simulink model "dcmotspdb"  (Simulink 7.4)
settings: Solver=ode15s  StartTime=0.0  StopTime=0.1  MaxStep=2e-5  RelTol=1e-5

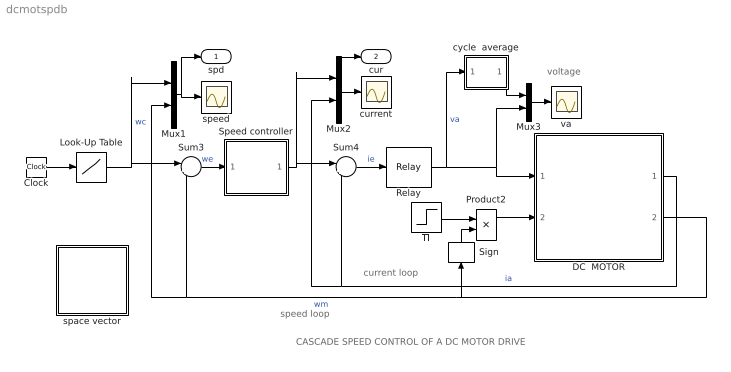
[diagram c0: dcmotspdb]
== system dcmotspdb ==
  note: voltage
  note: speed loop
  note: current loop
  note: CASCADE SPEED CONTROL OF A DC MOTOR DRIVE
  Clock : Clock
  DC  MOTOR : Subsystem  mask{Ra=2, La=0.0052, J=1.5e-4, Bm=1e-3, K=0.1}
      mask prompts: Ra "Armature resistance [ohm]"; La "Armature inductance [H]"; J "Moment of inertia [Kg.m^2]"; Bm "Frictional torque cefficient"; K "Electromechanical coupling coefficient [N.m/A]"
      mask help: Dynamic model of a dc motor
  Look-Up Table : Lookup  InputValues=[0 .03 .03 .08]  Table=[100 100 -100 -100]  OutDataType=sfix(16)  OutScaling=2^0
  Mux1 : Mux  Inputs=2
  Mux2 : Mux  Inputs=2
  Mux3 : Mux  Inputs=2
  Product2 : Product  OutDataType=sfix(16)  OutScaling=2^0
  Relay : Relay  OnSwitchValue=2  OffSwitchValue=-2  OnOutputValue=60  OffOutputValue=-60  OutDataType=sfix(16)  OutScaling=2^0
  Sign : Signum
  Speed controller : Subsystem  mask{Kp=1.5, Ki=650, sat=18}
      mask prompts: Kp "Proportional gain (Kp)"; Ki "Integral gain (Ki)"; sat "Saturation limit [pu]"
      mask help: Proportional-Integral Speed Controller
  Sum3 : Sum  Inputs=|+-  OutDataType=sfix(16)  OutScaling=2^0
  Sum4 : Sum  Inputs=|+-  OutDataType=sfix(16)  OutScaling=2^0
  Tl : Step  Time=0.07  SampleTime=0
  current : Scope
  cycle  average : Subsystem
  space vector : Subsystem
  speed : Scope
  va : Scope
  spd : Outport
  cur : Outport  Port=2
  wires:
  Mux1/1 -> speed/1, spd/1
  Mux2/1 -> current/1, cur/1
  Look-Up Table/1 -> Sum3/1, Mux1/1  "wc"
  Sum3/1 -> Speed controller/1(we)  "we"
  Sum4/1 -> Relay/1  "ie"
  Relay/1 -> cycle  average/1(sig), DC  MOTOR/1(va), Mux3/2  "va"
  Clock/1 -> Look-Up Table/1
  Speed controller/1(ic) -> Sum4/1, Mux2/1
  DC  MOTOR/2(wm) -> Sum3/2, Mux1/2, Sign/1  "wm"
  Product2/1 -> DC  MOTOR/2(Tl)
  Tl/1 -> Product2/1
  Sign/1 -> Product2/2
  DC  MOTOR/1(ia) -> Sum4/2, Mux2/2  "ia"
  Mux3/1 -> va/1
  cycle  average/1(ave) -> Mux3/1

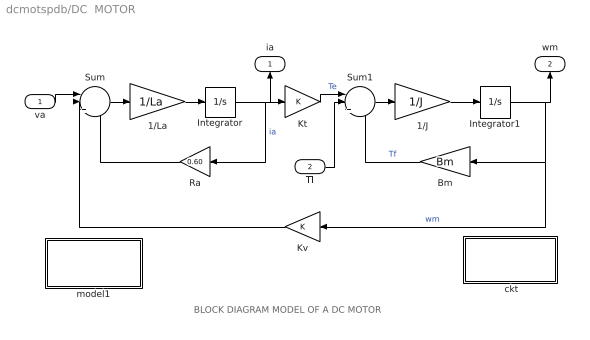
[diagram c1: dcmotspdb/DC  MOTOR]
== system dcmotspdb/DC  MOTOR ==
  note: BLOCK DIAGRAM MODEL OF A DC MOTOR
  va : Inport  OutDataType=sfix(16)  OutScaling=2^0
  Tl : Inport  Port=2  OutDataType=sfix(16)  OutScaling=2^0
  " ckt" : Subsystem
  1/J : Gain  Gain=1/J  ParameterDataType=sfix(16)  ParameterScaling=2^0  OutDataType=sfix(16)  OutScaling=2^0
  1/La : Gain  Gain=1/La  ParameterDataType=sfix(16)  ParameterScaling=2^0  OutDataType=sfix(16)  OutScaling=2^0
  Bm : Gain  Gain=Bm  ParameterDataType=sfix(16)  ParameterScaling=2^0  OutDataType=sfix(16)  OutScaling=2^0
  Integrator : Integrator
  Integrator1 : Integrator
  Kt : Gain  Gain=K  ParameterDataType=sfix(16)  ParameterScaling=2^0  OutDataType=sfix(16)  OutScaling=2^0
  Kv : Gain  Gain=K  ParameterDataType=sfix(16)  ParameterScaling=2^0  OutDataType=sfix(16)  OutScaling=2^0
  Ra : Gain  Gain=0.60  ParameterDataType=sfix(16)  ParameterScaling=2^0  OutDataType=sfix(16)  OutScaling=2^0
  Sum : Sum  Inputs=||+--  OutDataType=sfix(16)  OutScaling=2^0
  Sum1 : Sum  Inputs=||+--  OutDataType=sfix(16)  OutScaling=2^0
  model1 : Subsystem
  ia : Outport
  wm : Outport  Port=2
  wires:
  Kv/1 -> Sum/2
  Ra/1 -> Sum/3
  Kt/1 -> Sum1/1  "Te"
  Bm/1 -> Sum1/3  "Tf"
  Sum/1 -> 1/La/1
  1/La/1 -> Integrator/1
  Integrator/1 -> Ra/1, Kt/1, ia/1  "ia"
  Sum1/1 -> 1/J/1
  1/J/1 -> Integrator1/1
  Integrator1/1 -> Bm/1, Kv/1, wm/1  "wm"
  va/1 -> Sum/1
  Tl/1 -> Sum1/2

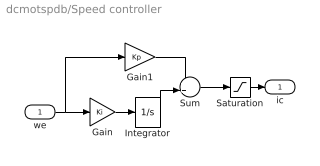
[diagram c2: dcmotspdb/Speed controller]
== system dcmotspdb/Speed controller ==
  we : Inport  OutDataType=sfix(16)  OutScaling=2^0
  Gain : Gain  Gain=Ki  ParameterDataType=sfix(16)  ParameterScaling=2^0  OutDataType=sfix(16)  OutScaling=2^0
  Gain1 : Gain  Gain=Kp  ParameterDataType=sfix(16)  ParameterScaling=2^0  OutDataType=sfix(16)  OutScaling=2^0
  Integrator : Integrator  LimitOutput=on  UpperSaturationLimit=sat  LowerSaturationLimit=-sat
  Saturation : Saturate  UpperLimit=sat  LowerLimit=-sat
  Sum : Sum  OutDataType=sfix(16)  OutScaling=2^0
  ic : Outport  InitialOutput=0
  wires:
  Saturation/1 -> ic/1
  Sum/1 -> Saturation/1
  Integrator/1 -> Sum/2
  we/1 -> Gain1/1, Gain/1
  Gain/1 -> Integrator/1
  Gain1/1 -> Sum/1

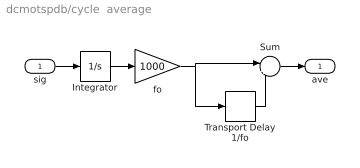
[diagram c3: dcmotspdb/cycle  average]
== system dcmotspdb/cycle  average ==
  sig : Inport  OutDataType=sfix(16)  OutScaling=2^0
  Integrator : Integrator
  Sum : Sum  Inputs=|+-  OutDataType=sfix(16)  OutScaling=2^0
  Transport Delay 1/fo : TransportDelay  DelayTime=1/1000
  fo : Gain  Gain=1000  ParameterDataType=sfix(16)  ParameterScaling=2^0  OutDataType=sfix(16)  OutScaling=2^0
  ave : Outport
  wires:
  Integrator/1 -> fo/1
  fo/1 -> Sum/1, Transport Delay 1/fo/1
  sig/1 -> Integrator/1
  Transport Delay 1/fo/1 -> Sum/2
  Sum/1 -> ave/1

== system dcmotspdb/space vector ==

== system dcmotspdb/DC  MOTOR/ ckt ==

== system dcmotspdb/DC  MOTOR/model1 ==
  note: Electrical system equation: va = Ra.ia + La.dia/dt + ea where ea = K.wm Mechanical system equation: Te = J.dwm/dt + Tl.signum(wm) + f(wm) where Te = K.ia
  note: Mathematical model of the dc machine
